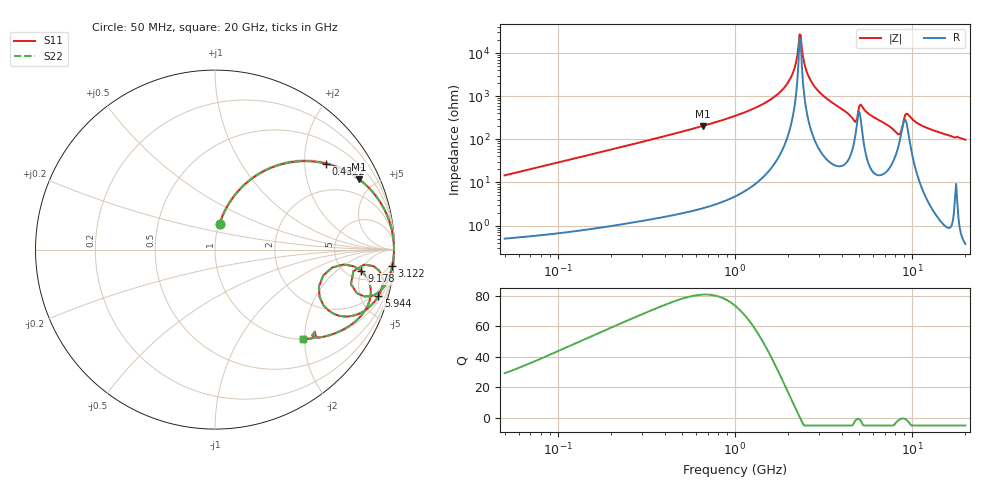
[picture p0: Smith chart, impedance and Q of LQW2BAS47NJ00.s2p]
!Murata Part Number: LQW2BAS47NJ00
!These Parameters are Measured in Series Mode Connection
!  o--[Z]--o
!Port1  Port2
!  o-------o
!Freq. Start=50[MHz] Stop=20[GHz], 401[Steps]
# Hz S RI R 50
!Freq.(Hz) S11(Real) S11(Imag) S21(Real) S21(Imag) S12(Real) S12(Imag) S22(Real) S22(Imag)
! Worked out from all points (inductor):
!   401 points, 50 MHz to 20 GHz, reference 50 ohm
!   read as one part in series: L = 46.2 nH near 51.52 MHz
!   highest Q = 80.9 at 657.4 MHz (marker M1), where L = 49.3 nH
!   self-resonance near 2.314 GHz
!   S11 on the Smith chart (normalised r, x): 50 MHz: 1.01, +0.29; 432.2 MHz: 1.03, +2.56; 3.122 GHz: 2, -21; 5.944 GHz: 1.37, -6.86; 9.178 GHz: 6.68, -4.94; 20 GHz: 1.01, -1.96
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5e7  0.0254 0.1413  0.9746 -0.1413  0.9746 -0.1413  0.0254 0.1413
1.364002e8  0.1398 0.3371  0.8602 -0.3371  0.8602 -0.3371  0.1398 0.3371
3.721004e8  0.544 0.4912  0.456 -0.4912  0.456 -0.4912  0.544 0.4912
4.322267e8  0.6197 0.4789  0.3803 -0.4789  0.3803 -0.4789  0.6197 0.4789
6.574395e8  0.8029 0.3917  0.1971 -0.3917  0.1971 -0.3917  0.8029 0.3917
1e9  0.9208 0.2633  0.0792 -0.2633  0.0792 -0.2633  0.9208 0.2633
1.476162e9  0.977 0.1398  0.023 -0.1398  0.023 -0.1398  0.977 0.1398
1.875929e9  0.9927 0.0662  0.00726 -0.0662  0.00726 -0.0662  0.9927 0.0662
2.114743e9  0.9962 0.0297  0.00377 -0.0297  0.00377 -0.0297  0.9962 0.0297
2.313601e9  0.997 0.00222  0.00297 -0.00222  0.00297 -0.00222  0.997 0.00222
2.383959e9  0.9969 -0.00699  0.00305 0.00699  0.00305 0.00699  0.9969 -0.00699
2.531158e9  0.9962 -0.0256  0.00377 0.0256  0.00377 0.0256  0.9962 -0.0256
2.728004e9  0.9943 -0.0491  0.00574 0.0491  0.00574 0.0491  0.9943 -0.0491
3.121702e9  0.9873 -0.093  0.0127 0.093  0.0127 0.093  0.9873 -0.093
4.677679e9  0.8307 -0.2602  0.1693 0.2602  0.1693 0.2602  0.8307 -0.2602
5.117541e9  0.914 -0.1167  0.086 0.1167  0.086 0.1167  0.914 -0.1167
5.944466e9  0.9099 -0.2605  0.0901 0.2605  0.0901 0.2605  0.9099 -0.2605
7.442007e9  0.7759 -0.3666  0.2241 0.3666  0.2241 0.3666  0.7759 -0.3666
8.389408e9  0.5824 -0.2633  0.4176 0.2633  0.4176 0.2633  0.5824 -0.2633
9.178299e9  0.8159 -0.1185  0.1841 0.1185  0.1841 0.1185  0.8159 -0.1185
1.183995e10  0.7798 -0.4017  0.2202 0.4017  0.2202 0.4017  0.7798 -0.4017
2e10  0.4903 -0.498  0.5097 0.498  0.5097 0.498  0.4903 -0.498
